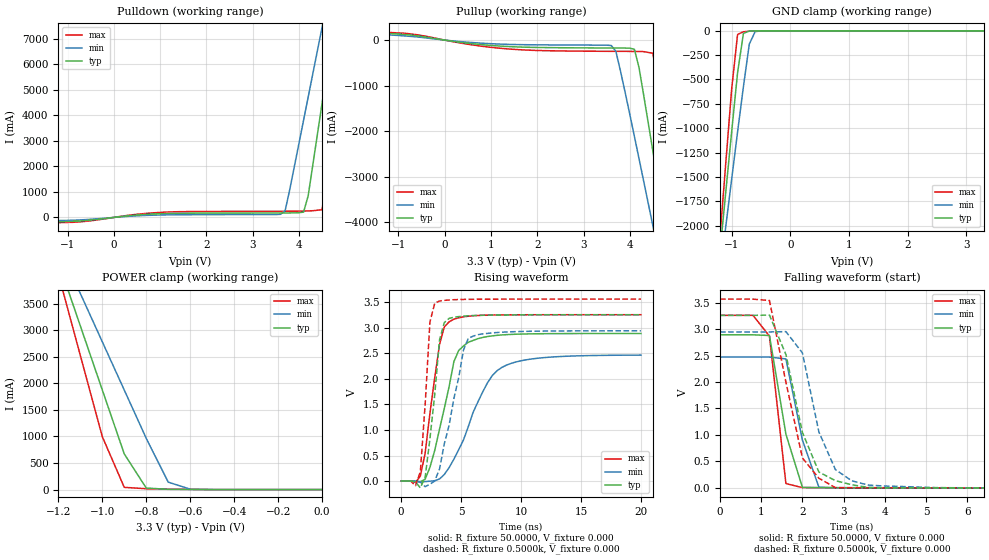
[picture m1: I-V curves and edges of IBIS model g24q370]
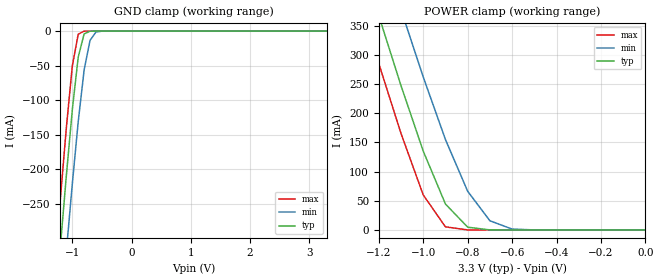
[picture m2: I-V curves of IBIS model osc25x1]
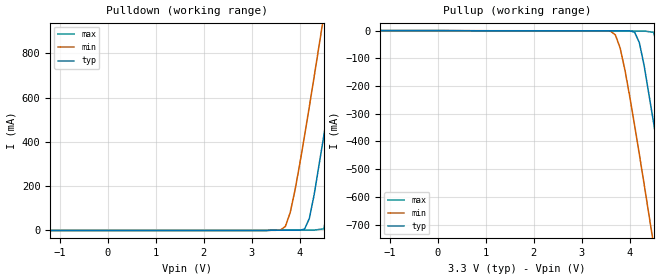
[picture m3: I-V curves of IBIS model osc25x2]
|   National Semiconductor Corporation
|   Interface Products Group
|   IBIS Model of DP83848 AspenPHY
|   48L LQFP Package
[IBIS Ver]   4.2
[Comment char]  |_char
[File name]   dp83848.ibs
[File Rev]   1.1
[Date]   9/01/2010
[Source]   File originated at National Semiconductor Corporation.
   Interface Group/Analog Division. All models created with
   Spectre s2ibis simulations by Sida Zhang.
   Originally Created on 8/24/2005 by Sida Zhang, modified
   on 9/01/2010 by Peggy Alavi
| All models created by s2ibis2 version 1.1
| North Carolina State University Electronics Research Laboratory  1995
[Notes]
   Rev 1.0 The file does not have TD+/TD- and RD+/RD- models
   due to the IBIS modeling limitations and design complexity.
   Rev 1.1 removes model selector. Model selector included a
   production test mode which is not available in the final
   product.
Begin IBIS Parser Results
| Do NOT edit this section manually!
Checking ...\dp83848.ibs for IBIS 4.2 Compatibility...
WARNING - Model osc25x1: POWER Clamp : Typical value never becomes zero
WARNING - Model osc25x1: POWER Clamp : Minimum value never becomes zero
WARNING - Model osc25x1: POWER Clamp : Maximum value never becomes zero
Errors  : 0
Warnings: 3
File Passed
| End IBIS Parser Results
[Disclaimer]
(C) Copyright National Semiconductor Corporation 2010
   All rights reserved
   National Semiconductor Corporation hereby grants
the user of this IBIS model a non-exclusive, nontransferable
license to use this IBIS model under the following terms.
Before using this IBIS model, the user should read this
license.  If the user does not accept these terms,  the
IBIS model should be returned to National within 30 days.
   The user is granted this license only to use the
IBIS model and is not granted rights to sell, load, rent,
lease or license the IBIS model in whole or in part, or in
modified form to anyone other than user. User may modify
the IBIS model to suit its specific applications but rights
to derivative works and such modifications shall belong to
National.
   This IBIS model is provided on an "AS IS" basis and
National makes absolutely no warranty with respect to the
information contained herein.NATIONAL DISCLAIMS AND CUSTOMER
WAIVES ALL WARRANTIES, EXPRESS OR IMPLIED, INCLUDING
WARRANTIES OF MERCHANTABILITY OR FITNESS FOR A PARTICULAR
PURPOSE. The entire risk as to quality and performance is
with the Customer. ACCORDINGLY, IN NO EVENT SHALL THE
COMPANY BE LIABLE FOR ANY DAMAGES, WHETHER IN CONTRACT OR
TORT,INCLUDING ANY LOST PROFITS OR OTHER INCIDENTAL,
CONSEQUENTIAL, EXEMPLARY, OR PUNITIVE DAMAGES ARISING OUT
OF THE USE OR APPLICATION OF THE IBIS model provided in
this package.Further, National reserves the right to make
changes without notice to any product herein to improve
reliability, function, or design. National does not convey
any license under patent rights or any other intellectual
property rights, including those of third parties.
   National is not obligated to provide maintenance or support
for the licensed IBIS model.
[Copyright]   Copyright 2010, National Semiconductor, All Rights Reserved
[Component]   DP83848
[Manufacturer]  National Semiconductor Corporation
[Package]
|   typ   min   max
R_pkg   50.0m   50.0m   50.0m
L_pkg   1.88nH   1.7922n   2.11433n
C_pkg   0.306pF   0.27505p   0.33960p
[Pin]   signal_name   model_name   R_pin   L_pin   C_pin
1   TX_CLK   g24q370   50.0m   2.11433n   0.27505p
2   TX_EN   g24q370   50.0m   2.01554n   0.33960p
3   TXD_0   g24q370   50.0m   1.94357n   0.32802p
4   TXD_1   g24q370   50.0m   1.89274n   0.32012p
5   TXD_2   g24q370   50.0m   1.83759n   0.31097p
6   TXD_3/SNI_MODE   g24q370   50.0m   1.79220n   0.30663p
7   PWR_DOWN/INT   g24q370   50.0m   1.79220n   0.30663p
8   TCK   g24q370   50.0m   1.83759n   0.31097p
9   TDO   g24q370   50.0m   1.89274n   0.32012p
10   TMS   g24q370   50.0m   1.94357n   0.32802p
11   TRST#   g24q370   50.0m   2.01554n   0.33960p
12   TDI   g24q370   50.0m   2.11433n   0.27505p
13   RD-   NC   50.0m   2.11433n   0.27505p
14   RD+   NC   50.0m   2.01554n   0.33960p
15   AGND   GND   50.0m   1.94357n   0.32802p
16   TD-   NC   50.0m   1.89274n   0.32012p
17   TD+   NC   50.0m   1.83759n   0.31097p
18   PFBIN1   NC   50.0m   1.79220n   0.30663p
19   AGND   GND   50.0m   1.79220n   0.30663p
20   RESERVED   NC   50.0m   1.83759n   0.31097p
21   RESERVED   NC   50.0m   1.89274n   0.32012p
22   AVDD33   POWER   50.0m   1.94357n   0.32802p
23   PFBOUT   NC   50.0m   2.01554n   0.33960p
24   RBIAS   NC   50.0m   2.11433n   0.27505p
25   25MHz_OUT   g24q370   50.0m   2.11433n   0.27505p
26   LED_ACT/COL/AN_EN   g24q370   50.0m   2.01554n   0.33960p
27   LED_SPEED/AN1   g24q370   50.0m   1.94357n   0.32802p
28   LED_LINK/AN0   g24q370   50.0m   1.89274n   0.32012p
29   RESET_N   g24q370   50.0m   1.83759n   0.31097p
30   MDIO   g24q370   50.0m   1.79220n   0.30663p
31   MDC   g24q370   50.0m   1.79220n   0.30663p
32   IOVDD33   POWER   50.0m   1.83759n   0.31097p
33   X2   osc25x2   50.0m   1.89274n   0.32012p
34   X1   osc25x1   50.0m   1.94357n   0.32802p
35   IOGND   GND   50.0m   2.01554n   0.33960p
36   DGND   GND   50.0m   2.11433n   0.27505p
37   PFBIN2   NC   50.0m   2.11433n   0.27505p
38   RX_CLK   g24q370   50.0m   2.01554n   0.33960p
39   RX_DV/MII_MODE   g24q370   50.0m   1.94357n   0.32802p
40   CRS/CRS_DV/LED_CFG  g24q370   50.0m   1.89274n   0.32012p
41   RX_ER/MDIX_EN   g24q370   50.0m   1.83759n   0.31097p
42   COL/PHYAD0   g24q370   50.0m   1.79220n   0.30663p
43   RXD_0/PHYAD1   g24q370   50.0m   1.79220n   0.30663p
44   RXD_1/PHYAD2   g24q370   50.0m   1.83759n   0.31097p
45   RXD_2/PHYAD3   g24q370   50.0m   1.89274n   0.32012p
46   RXD_3/PHYAD4   g24q370   50.0m   1.94357n   0.32802p
47   IOGND   GND   50.0m   2.01554n   0.33960p
48   IOVDD33   POWER   50.0m   2.11433n   0.27505p
| Models and submodels in the file (3): g24q370 (I/O), osc25x1 (Input), osc25x2 (Output)
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|[Diff_pin]   inv_pin   vdiff   tdelay_typ   tdelay_min   tdelay_max
| The '+' pin is Diff_pin and the '-' pin is the inv_pin
|14   13   0.100   0 0 0
|17   16   0.100   0 0 0
|   Model g24q370
[Model]   g24q370
Model_type   I/O
Polarity   Non-Inverting
Enable   Active-High
Vinl = 0.8000V
Vinh = 2.0000V
Vmeas = 1.5000V
C_comp   1.0640pF   1.0620pF   1.0670pF
[Temperature Range]   25.0000   0.1250k   -40.0000
[Voltage Range]   3.3000V   3.0000V   3.6000V
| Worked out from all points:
|   slope of the pulldown table from 0 to 0.495 V, typ, clamps not added: 5.31 ohm
|   slope of the pullup table from 0 to 0.495 V, typ, clamps not added: 7.25 ohm
|   GND clamp passes 1 mA (typ) near -0.64 V on its own axis
|   POWER clamp passes 1 mA (typ) near -0.54 V on its own axis
|   rising waveform, R_fixture 50.0000, V_fixture 0.000: 20-80 % time 1.6ns typ, 2.8ns min, 1.1ns max; typ from 0 V to 2.89 V
|   rising waveform, R_fixture 0.5000k, V_fixture 0.000: 20-80 % time 833ps typ, 1.56ns min, 573ps max; typ from 0 V to 3.26 V
|   falling waveform, R_fixture 50.0000, V_fixture 0.000: 20-80 % time 452ps typ, 464ps min, 281ps max; typ from 2.89 V to 0 V
|   falling waveform, R_fixture 0.5000k, V_fixture 0.000: 20-80 % time 659ps typ, 611ps min, 580ps max; typ from 3.26 V to 0 V
[Pulldown]
| voltage   I(typ)   I(min)   I(max)
-3.3V     -160.5mA   -118.3mA   -200.7mA
-900mV    -153.7mA   -111mA     -192.4mA
1.1V      151.8mA    98.11mA    206.2mA
3.6V      174.1mA    121.6mA    241.2mA
3.7V      174.7mA    254.1mA    242mA
4.1V      208.2mA    3.809A     248.7mA
4.2V      852.2mA    4.721A     254.3mA
4.5V      4.477A     7.457A     302mA
4.7V      6.898A     9.283A     2.796A
4.9V      9.321A     11.11A     5.87A
5.1V      11.75A     12.94A     8.947A
6.6V      30.05A     26.73A     32.17A
[Pullup]
| voltage   I(typ)   I(min)   I(max)
-3.3V     188.1mA    165.2mA    206.9mA
-900mV    123.6mA    93.95mA    153.1mA
1.3V      -138.1mA   -91.87mA   -188.7mA
3.6V      -174.3mA   -119.7mA   -247.2mA
3.7V      -174.6mA   -248.3mA   -247.7mA
4.1V      -202.3mA   -2.118A    -249.5mA
4.2V      -607mA     -2.608A    -250.6mA
4.5V      -2.447A    -4.087A    -288.9mA
4.7V      -3.699A    -5.076A    -1.602A
4.9V      -4.956A    -6.068A    -3.14A
5.1V      -6.215A    -7.061A    -4.687A
6.6V      -15.68A    -14.52A    -16.34A
[GND_clamp]
| voltage   I(typ)   I(min)   I(max)
-3.3V     -15.47A    -12.9A     -18.37A
-1.2V     -2.269A    -2.494A    -2.116A
-1.1V     -1.647A    -2.005A    -1.349A
-1V       -1.031A    -1.519A    -592.6mA
-900mV    -430.7mA   -1.039A    -37.49mA
-800mV    -26.32mA   -572.9mA   -9.444mA
-700mV    -1.926mA   -136.4mA   -3.598mA
-600mV    -247.7uA   -8.119mA   -648.8uA
-400mV    -1.571uA   -27.47uA   -1.62uA
3.3V      22.02pA    3.648uA    15.2pA
[POWER_clamp]
| voltage   I(typ)   I(min)   I(max)
-3.3V     29.64A     23.74A     36.19A
-1.2V     4.29A      4.604A     4.058A
-1.1V     3.083A     3.693A     2.528A
-1V       1.877A     2.784A     997.8mA
-900mV    671.8mA    1.874A     42.61mA
-800mV    29.37mA    964.9mA    16.3mA
-700mV    5.409mA    140.5mA    9.688mA
-600mV    1.864mA    8.479mA    4.466mA
0V        22.02pA    589.3pA    18.15pA
[Ramp]
| variable   typ   min   max
dV/dt_r   1.7348/1.6680n   1.4811/3.0471n   1.9560/1.1060n
dV/dt_f   1.8068/1.8411n   1.5594/3.2593n   2.0132/1.2189n
R_load = 50.0000
[Rising Waveform]
R_fixture = 50.0000
V_fixture = 0.000
V_fixture_min = 0.000
V_fixture_max = 0.000
| time   V(typ)   V(min)   V(max)
0s        121pV      6.465nV    36.64pV
1.6ns     -12.04mV   -15.26mV   96.9mV
2ns       34.22mV    -11.2mV    543.1mV
2.4ns     268mV      -3.569mV   1.326V
3.2ns     1.016V     39.7mV     2.674V
4ns       1.85V      262mV      3.12V
4.8ns     2.559V     613.5mV    3.2V
7.2ns     2.832V     1.925V     3.252V
8.4ns     2.864V     2.227V     3.257V
20ns      2.891V     2.468V     3.26V
[Rising Waveform]
R_fixture = 0.5000k
V_fixture = 0.000
V_fixture_min = 0.000
V_fixture_max = 0.000
| time   V(typ)   V(min)   V(max)
0s        130pV      7.171nV    38.79pV
1.2ns     -20.26mV   28.89uV    -92.41mV
1.6ns     -134.2mV   -21.16mV   180.7mV
2ns       72.06mV    -111.1mV   1.492V
2.4ns     825.8mV    -63.59mV   3.114V
2.8ns     1.692V     781.9uV    3.485V
3.2ns     2.765V     233.9mV    3.529V
3.6ns     3.107V     729.7mV    3.542V
5.6ns     3.239V     2.796V     3.562V
20ns      3.259V     2.945V     3.566V
[Falling Waveform]
R_fixture = 50.0000
V_fixture = 0.000
V_fixture_min = 0.000
V_fixture_max = 0.000
| time   V(typ)   V(min)   V(max)
0s        2.891V     2.471V     3.26V
800ps     2.891V     2.471V     3.26V
1.2ns     2.878V     2.471V     2.867V
1.6ns     1.014V     2.436V     81.31mV
2ns       8.918mV    903.1mV    5.147mV
2.4ns     3.412mV    11.78mV    4.297mV
20ns      2.471uV    23.79uV    19.15uV
[Falling Waveform]
R_fixture = 0.5000k
V_fixture = 0.000
V_fixture_min = 0.000
V_fixture_max = 0.000
| time   V(typ)   V(min)   V(max)
0s        3.259V     2.945V     3.566V
1.2ns     3.265V     2.946V     3.539V
1.6ns     2.519V     2.952V     1.996V
2ns       1.048V     2.55V      564.1mV
2.4ns     298.8mV    1.056V     181.6mV
2.8ns     136.3mV    345.2mV    4.978mV
3.2ns     58.01mV    132.1mV    1.436mV
3.6ns     8.285mV    52.25mV    931.6uV
5.2ns     739.4uV    5.88mV     479.6uV
20ns      3.35uV     19.65uV    13.62uV
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|   Model osc25x1
[Model]   osc25x1
Model_type   Input
Polarity   Inverting
Enable   Active-High
Vinl = 0.8000V
Vinh = 2.0000V
C_comp   1.0000pF   1.0000pF   1.0000pF
[Temperature Range]   25.0000   0.1250k   -40.0000
[Voltage Range]   3.3000V   3.0000V   3.6000V
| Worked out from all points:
|   GND clamp passes 1 mA (typ) near -0.72 V on its own axis
|   POWER clamp passes 1 mA (typ) near -0.72 V on its own axis
[GND_clamp]
| voltage   I(typ)   I(min)   I(max)
-3.3V     -2.622A    -2.694A    -2.579A
-1.3V     -414.8mA   -523mA     -346.4mA
-1.2V     -310.3mA   -419.8mA   -240.9mA
-1.1V     -208.9mA   -318.8mA   -139.7mA
-1V       -114.1mA   -221.5mA   -50.66mA
-900mV    -37.58mA   -131mA     -4.515mA
-800mV    -4.019mA   -56.03mA   -47.48uA
-700mV    -108.1uA   -13.33mA   -2.355uA
-600mV    -3.685uA   -1.282mA   -1.753uA
-400mV    -1.001uA   -4.899uA   -1.167uA
3.3V      8.25uA     7.477uA    9.629uA
[POWER_clamp]
| voltage   I(typ)   I(min)   I(max)
-3.3V     3.1A       3.186A     3.05A
-1.3V     490.5mA    618.5mA    409.7mA
-1.2V     366.9mA    496.4mA    284.9mA
-1.1V     247mA      377mA      165.2mA
-1V       135mA      261.9mA    59.9mA
-900mV    44.44mA    154.8mA    5.346mA
-800mV    4.759mA    66.25mA    66.21uA
-700mV    135.7uA    15.76mA    12.92uA
-600mV    12.33uA    1.522mA    12.26uA
-500mV    9.553uA    95.08uA    11.96uA
0V        8.25uA     6.563uA    10.5uA
|   Model osc25x2
[Model]   osc25x2
Model_type   Output
Polarity   Inverting
Enable   Active-High
Vmeas = 1.5000V
C_comp   1.0000pF   1.0000pF   1.0000pF
[Temperature Range]   25.0000   0.1250k   -40.0000
[Voltage Range]   3.3000V   3.0000V   3.6000V
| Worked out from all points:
|   slope of the pullup table from 0 to 0.495 V, typ, clamps not added: 1.19 kohm
[Pulldown]
| voltage   I(typ)   I(min)   I(max)
-3.3V     0A         0A         0A
3.6V      1.099mA    2.318mA    1.555mA
3.7V      1.103mA    18.37mA    1.56mA
3.8V      1.11mA     80.08mA    1.567mA
4.1V      6.217mA    428mA      1.603mA
4.2V      54.57mA    559.8mA    1.639mA
4.5V      425.9mA    967.9mA    7.417mA
4.7V      707.9mA    1.245A     200.5mA
4.9V      996mA      1.525A     486.1mA
5.1V      1.287A     1.806A     783.4mA
5.3V      1.58A      2.089A     1.085A
6.6V      3.503A     3.939A     3.076A
[Pullup]
| voltage   I(typ)   I(min)   I(max)
-3.3V     0A         0A         0A
3.6V      -1.081mA   -2.06mA    -1.527mA
3.7V      -1.083mA   -15.55mA   -1.53mA
3.8V      -1.086mA   -63.14mA   -1.534mA
4.1V      -5.367mA   -340.7mA   -1.543mA
4.2V      -43.48mA   -446.6mA   -1.551mA
4.5V      -335.7mA   -775mA     -6.395mA
4.7V      -559.6mA   -998.5mA   -156mA
4.9V      -788.6mA   -1.224A    -379.2mA
5.1V      -1.02A     -1.451A    -612.3mA
5.3V      -1.253A    -1.678A    -849mA
6.6V      -2.784A    -3.17A     -2.413A
[Ramp]
| variable   typ   min   max
dV/dt_r   1.7737/0.4988n   1.5328/0.7567n   1.9870/0.3615n
dV/dt_f   1.8364/0.4766n   1.5967/0.7630n   2.0404/0.3438n
R_load = 10.0000k
